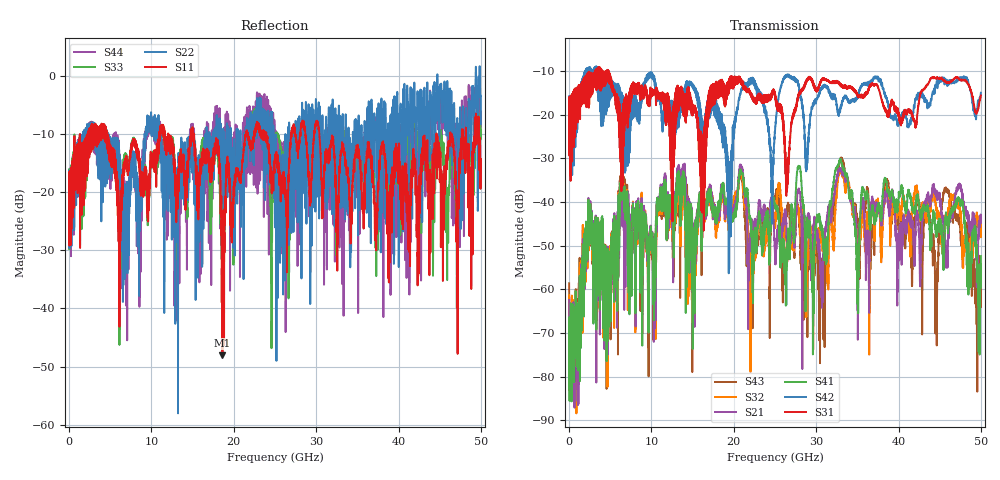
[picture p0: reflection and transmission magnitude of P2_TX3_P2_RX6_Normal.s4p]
!Keysight Technologies,N5225B,MY57041031,A.13.20.10
!Date: Friday, May 31, 2019 11:36:00
!Correction: S11(Full 4 Port(1,2,3,4))
!S12(Full 4 Port(1,2,3,4))
!S13(Full 4 Port(1,2,3,4))
!S14(Full 4 Port(1,2,3,4))
!S21(Full 4 Port(1,2,3,4))
!S22(Full 4 Port(1,2,3,4))
!S23(Full 4 Port(1,2,3,4))
!S24(Full 4 Port(1,2,3,4))
!S31(Full 4 Port(1,2,3,4))
!S32(Full 4 Port(1,2,3,4))
!S33(Full 4 Port(1,2,3,4))
!S34(Full 4 Port(1,2,3,4))
!S41(Full 4 Port(1,2,3,4))
!S42(Full 4 Port(1,2,3,4))
!S43(Full 4 Port(1,2,3,4))
!S44(Full 4 Port(1,2,3,4))
!S4P File: Measurements: <S11,S12,S13,S14>,
!<S21,S22,S23,S24>,
!<S31,S32,S33,S34>,
!<S41,S42,S43,S44>:
# Hz S  dB  R 50.0
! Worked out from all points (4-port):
!   5000 points, 10 MHz to 50 GHz, reference 50 ohm
!   strongest paths, dB at 10 MHz, 12.51 GHz, 25.01 GHz, 37.51 GHz, 50 GHz:
!     S31: -19.6, -42.7, -16.1, -13.6, -15.6
!     S42: -19.4, -16.8, -23.7, -11.3, -14.9
!     S41: -79.6, -40.1, -40.6, -41.0, -52.4
!     S21: -62.4, -42.7, -52.6, -41.1, -44.6
!     S32: -61.4, -45.4, -44.0, -40.0, -45.5
!     S43: -58.6, -42.4, -38.8, -40.3, -56.5
!   lowest |S11| = -48.1 dB at 18.62 GHz (marker M1), VSWR 1.01, Z = 49.7 - j0.286 ohm
!   |S11| at or under -10 dB: 4.63 GHz to 10.95 GHz (6.317 GHz wide, 81.1 % of centre); 15.14 GHz to 21.46 GHz (6.325 GHz wide, 34.6 % of centre); 30.38 GHz to 44.61 GHz (14.23 GHz wide, 37.9 % of centre)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
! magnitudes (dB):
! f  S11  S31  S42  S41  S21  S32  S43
! 10 MHz  -19.6  -19.6  -19.4  -79.6  -62.4  -61.4  -58.6
! 2.5 GHz  -13.4  -15.8  -11.4  -43.4  -43.2  -44.0  -44.2
! 18.62 GHz  -48.1  -12.3  -23.1  -36.4  -37.8  -38.6  -37.0
! 30.59 GHz  -15.4  -12.4  -14.2  -46.4  -54.4  -47.6  -54.9
! 33.03 GHz  -13.4  -13.4  -17.8  -30.5  -32.5  -32.8  -29.8
! 45.81 GHz  -14.0  -12.6  -12.4  -44.1  -53.3  -44.2  -37.0
! 50 GHz  -15.3  -15.6  -14.9  -52.4  -44.6  -45.5  -56.5
